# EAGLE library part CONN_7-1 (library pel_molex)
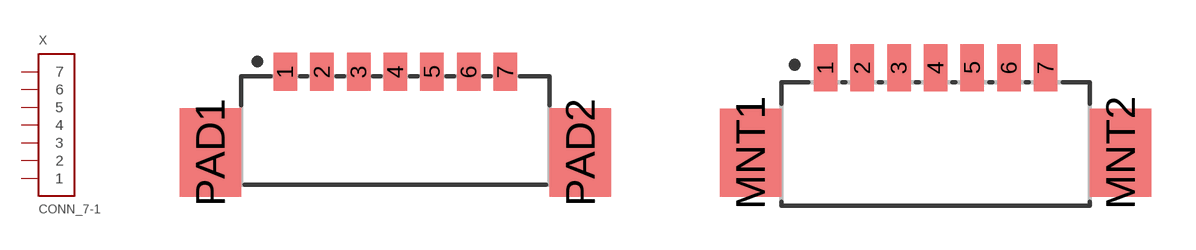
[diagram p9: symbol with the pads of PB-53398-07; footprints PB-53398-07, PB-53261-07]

Designator prefix X

## CONN_7-1-53398  [PB-53398-07]
1  1
2  2
3  3
4  4
5  5
6  6
7  7

## CONN_7-1-53261  [PB-53261-07]
Pads as for PB-53398-07

## CONN_7-1-53047  [PB-53047-07]
Pads as for PB-53398-07

## CONN_7-1-502386  [CM-502386-07]
Pads as for PB-53398-07

## CONN_7-1-502382  [CM-502382-07]
Pads as for PB-53398-07

## Footprint PB-53398-07 (pad centres in mm)
smd 0.8 x 1.3: 1 -3.75,1.25; 2 -2.5,1.25; 3 -1.25,1.25; 4 0,1.25; 5 1.25,1.25; 6 2.5,1.25; 7 3.75,1.25
smd 2.1 x 3: PAD1 -6.3,-1.5; PAD2 6.3,-1.5

## Footprint PB-53261-07 (pad centres in mm)
smd 0.8 x 1.6: 1 -3.75,1.1; 2 -2.5,1.1; 3 -1.25,1.1; 4 0,1.1; 5 1.25,1.1; 6 2.5,1.1; 7 3.75,1.1
smd 2.1 x 3: MNT1 -6.3,-1.8; MNT2 6.3,-1.8

## Footprint PB-53047-07 (pad centres in mm)
drill 0.5: 1 -3.75,0; 2 -2.5,0; 3 -1.25,0; 4 0,0; 5 1.25,0; 6 2.5,0; 7 3.75,0

## Footprint CM-502386-07 (pad centres in mm)
Click Mate Right Angle
smd 0.6 x 1.7: 1 3.75,-4.55; 2 2.5,-4.55; 3 1.25,-4.55; 4 0,-4.55; 5 -1.25,-4.55; 6 -2.5,-4.55; 7 -3.75,-4.55
smd 1 x 2.7: P1 5.6,-1.25; P2 -5.6,-1.25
